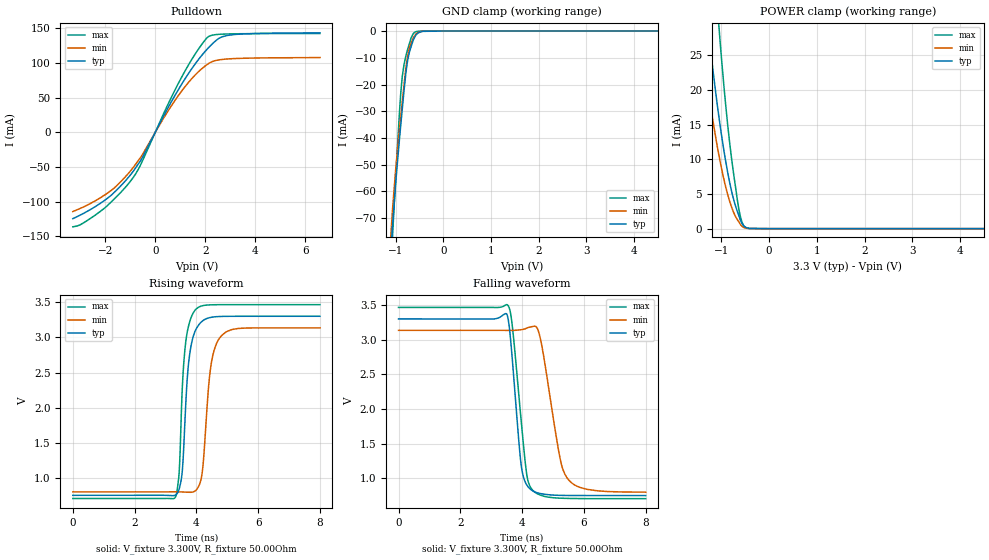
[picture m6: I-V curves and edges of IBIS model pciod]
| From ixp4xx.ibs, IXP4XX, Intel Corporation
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[Model]   pciod
Model_type   I/O_open_drain
Vinl = 800.000mV
Vinh = 2.000V
Vmeas = 1.500V
Cref = 0.000F
|   typ   min   max
C_comp   3.000pF   2.700pF   3.300pF
[Voltage Range]   3.300V   3.135V   3.465V
[Temperature Range]   25.0   110.0   -40.0
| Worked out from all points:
|   slope of the pulldown table from 0 to 0.495 V, typ, clamps not added: 14.5 ohm
|   GND clamp passes 1 mA (typ) near -0.55 V on its own axis
|   POWER clamp passes 1 mA (typ) near -0.59 V on its own axis
|   falling waveform, V_fixture 3.300V, R_fixture 50.00Ohm: 20-80 % time 283ps typ, 507ps min, 346ps max; typ from 3.3 V to 0.753 V
|   rising waveform, V_fixture 3.300V, R_fixture 50.00Ohm: 20-80 % time 224ps typ, 265ps min, 187ps max; typ from 0.753 V to 3.3 V
[Pulldown]
|   Voltage   I(typ)   I(min)   I(max)
-3.3V     -124.6mA   -114.4mA   -136.4mA
-2.99V    -119.2mA   -109.6mA   -133.2mA
-1.995V   -97.34mA   -89.79mA   -108.3mA
-1.605V   -85.39mA   -79.22mA   -94.97mA
-895mV    -56.88mA   -51.41mA   -65.85mA
-525mV    -37.09mA   -32.82mA   -42.22mA
940mV     62.44mA    53.71mA    71.6mA
1.535V    95.49mA    80.32mA    109.3mA
2.08V     120mA      97.84mA    136.7mA
2.545V    135.5mA    104.5mA    141.4mA
2.89V     139.8mA    105.8mA    141.9mA
6.595V    143.5mA    107.9mA    142.6mA
[GND Clamp]
|   Voltage   I(typ)   I(min)   I(max)
-3.3V     -1.837A    -1.782A    -2.142A
-1.125V   -89.61mA   -82.47mA   -99.52mA
-1.065V   -72.55mA   -66.27mA   -76.21mA
-995mV    -55.6mA    -50.79mA   -53mA
-910mV    -38.32mA   -34.82mA   -27.37mA
-860mV    -28.72mA   -26.04mA   -16.73mA
-790mV    -16.24mA   -14.37mA   -9.578mA
-750mV    -11.01mA   -9.296mA   -6.858mA
-675mV    -5.744mA   -4.387mA   -2.48mA
-580mV    -1.627mA   -1.201mA   -252.6uA
0V        -56.89nA   -17.57nA   -32.79pA
6.595V    0A         0A         0A
[POWER Clamp]
|   Voltage   I(typ)   I(min)   I(max)
-3.3V     221.1mA    178.3mA    345.2mA
-1.48V    42.85mA    30.79mA    74.12mA
-1.43V    39.23mA    27.99mA    68.17mA
-1.265V   28.16mA    19.53mA    49.72mA
-1.065V   16.76mA    11.05mA    30.24mA
-1.025V   14.78mA    9.615mA    26.79mA
-915mV    9.907mA    6.159mA    18.18mA
-780mV    5.204mA    2.981mA    9.739mA
-635mV    1.89mA     986.7uA    2.845mA
-570mV    776uA      354.8uA    984.2uA
-515mV    310.8uA    129.8uA    274uA
6.595V    0A         0A         0A
[Ramp]
R_load = 50.00Ohm
|   typ   min   max
dV/dt_r   1.394uV/11.871ps  461.970nV/281.651ps  56.121nV/8.965ps
dV/dt_f   1.528V/282.540ps   1.400V/505.797ps   1.654V/346.108ps
[Falling Waveform]
V_fixture = 3.300V
V_fixture_min = 3.135V
V_fixture_max = 3.465V
R_fixture = 50.00Ohm
|   Time   V(typ)   V(min)   V(max)
0s        3.3V       3.135V     3.465V
3.55ns    3.293V     3.134V     3.488V
3.69ns    2.679V     3.134V     3.171V
3.98ns    1.162V     3.145V     1.785V
4.18ns    887.1mV    3.173V     985.6mV
4.44ns    801.2mV    3.192V     793.1mV
4.65ns    777.7mV    2.885V     750.8mV
5.23ns    756.3mV    1.287V     715.8mV
5.45ns    754.7mV    1.012V     712.5mV
8ns       753.2mV    802.4mV    708.3mV
[Rising Waveform]
V_fixture = 3.300V
V_fixture_min = 3.135V
V_fixture_max = 3.465V
R_fixture = 50.00Ohm
|   Time   V(typ)   V(min)   V(max)
0s        753.2mV    802.4mV    708.3mV
3.32ns    756.2mV    803.2mV    725.8mV
3.44ns    840.8mV    802.9mV    1.068V
3.53ns    1.041V     801.4mV    2.137V
3.65ns    1.998V     798.7mV    2.914V
4.02ns    3.14V      843mV      3.413V
4.2ns     3.234V     1.118V     3.45V
4.47ns    3.284V     2.596V     3.463V
4.75ns    3.297V     2.99V      3.465V
8ns       3.3V       3.135V     3.465V
